(* Logix 5000 AddOnInstructionDefinition export Banner_QCM50_K1_PD_v4; software revision 33.00 *)

TYPE Banner_QCM50_K1_PDI_v4 :
STRUCT
   Signal_Quality : INT;   // 0 = no signal, 1 = overflow, 2 to 100.
   Switching_Quality : SINT;
   Q1 : SINT;
   PDI_DT : SINT[2];
END_STRUCT
END_TYPE

ADD_ON_INSTRUCTION Banner_QCM50_K1_PD_v4   (* revision 4.0, vendor Banner Engineering *)
VAR_IN_OUT
   PDI : Banner_QCM50_K1_PDI_v4; {required}
END_VAR
VAR_INPUT
   Byte_Swap : BOOL; {required}
   K : DINT; {required}
END_VAR
VAR
   Temp_Byte : SINT[6]; {access None}
END_VAR

ROUTINE Logic   (* ladder *)
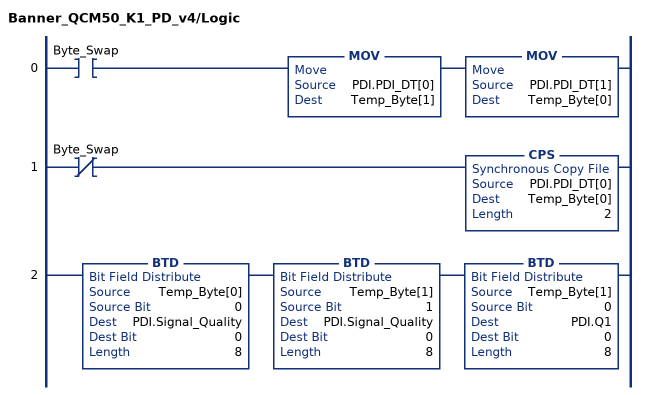
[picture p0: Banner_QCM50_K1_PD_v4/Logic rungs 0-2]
   0: XIC(Byte_Swap)MOV(PDI.PDI_DT[0],Temp_Byte[1])MOV(PDI.PDI_DT[1],Temp_Byte[0]);
   1: XIO(Byte_Swap)CPS(PDI.PDI_DT[0],Temp_Byte[0],2);
   2: BTD(Temp_Byte[0],0,PDI.Signal_Quality,0,8)BTD(Temp_Byte[1],1,PDI.Signal_Quality,0,8)BTD(Temp_Byte[1],0,PDI.Q1,0,8);
END_ROUTINE
END_ADD_ON_INSTRUCTION
